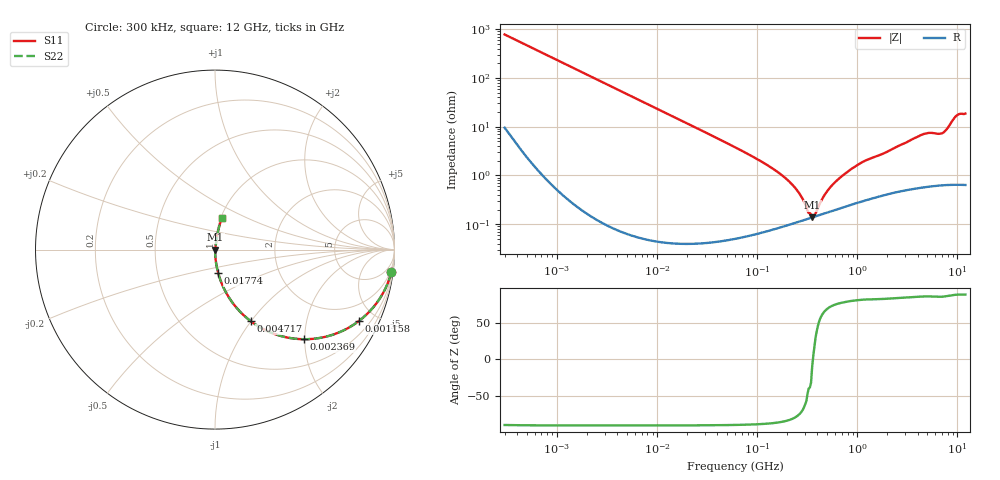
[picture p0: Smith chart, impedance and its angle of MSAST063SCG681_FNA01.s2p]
! MSAST063SCG681_FNA01  S-PARAMETER MODEL  ( General Type )
! Model Generated by TAIYO YUDEN Corporation (http://www.ty-top.com)
! Version 1.0
! TAIYO YUDEN Control No. 160830
! Copyright(c) 2016 TAIYO YUDEN CO.,LTD. All Rights Reserved.
! Product Description (link to TY-COMPAS)
! https://ds.yuden.co.jp/TYCOMPAS/or/detail?pn=MSAST063SCG681JFNA01&u=M
! Products Name : Multilayer Ceramic Capacitors
! Characteristics :
!  Capacitance : 680 pF , Rated Voltage : 25V , TCC : CG / C0G
!  Case Size : 0.6 x 0.3 / 0.024 x 0.012 [mm/inch] , Thickness : 0.3 / 0.012 [mm/inch]
!  (Conditions: Temperature = 25 degC , DC Bias Current/Voltage = 0A / 0V)
! External Node Assignments :
!  1  o---| |---o  2
! GND o---------o GND
! Frequency Range : 0.3MHz  -  12000MHz  [ 401 STEP ]
# MHz S RI R 50
! Freq[MHz].  S11 Real  S11 Imag  S21 Real  S21 Imag  S12 Real  S12 Imag  S22 Real  S22 Imag
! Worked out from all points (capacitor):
!   401 points, 300 kHz to 12 GHz, reference 50 ohm
!   read as one part in series: C = 680 pF near 316.3 kHz
!   lowest |Z| = 140 mohm at 354 MHz (marker M1)
!   series resonance near 360.2 MHz, so ESL is about 290 pH
!   S11 on the Smith chart (normalised r, x): 300 kHz: 1, -16; 1.158 MHz: 1.01, -4.04; 2.369 MHz: 1.00, -1.98; 4.717 MHz: 1.00, -0.99; 17.74 MHz: 1.00, -0.26; 12 GHz: 1.01, +0.37
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0.3  0.9823 -0.1257  0.0177 0.1257  0.0177 0.1257  0.9823 -0.1257
0.646801  0.9283 -0.2563  0.0717 0.2563  0.0717 0.2563  0.9283 -0.2563
1.158468  0.8028 -0.397  0.1972 0.397  0.1972 0.397  0.8028 -0.397
1.769972  0.636 -0.4804  0.364 0.4804  0.364 0.4804  0.636 -0.4804
2.36877  0.494 -0.4993  0.506 0.4993  0.506 0.4993  0.494 -0.4993
4.716902  0.1978 -0.3977  0.8022 0.3977  0.8022 0.3977  0.1978 -0.3977
10.44266  0.0481 -0.2131  0.9519 0.2131  0.9519 0.2131  0.0481 -0.2131
17.7384  0.0174 -0.1293  0.9826 0.1293  0.9826 0.1293  0.0174 -0.1293
60  0.00193 -0.0378  0.9981 0.0378  0.9981 0.0378  0.00193 -0.0378
197.6437  0.00101 -0.00825  0.999 0.00825  0.999 0.00825  0.00101 -0.00825
257.5933  0.00113 -0.00442  0.9989 0.00442  0.9989 0.00442  0.00113 -0.00442
335.7268  0.00133 -0.00105  0.9987 0.00105  0.9987 0.00105  0.00133 -0.00105
353.9943  0.00137 -0.000237  0.9986 0.000237  0.9986 0.000237  0.00137 -0.000237
383.2761  0.00145 0.000845  0.9985 -0.000845  0.9985 -0.000845  0.00145 0.000845
499.5319  0.00175 0.0044  0.9982 -0.0044  0.9982 -0.0044  0.00175 0.0044
668.5285  0.00218 0.00864  0.9978 -0.00864  0.9978 -0.00864  0.00218 0.00864
1105.905  0.00324 0.0181  0.9968 -0.0181  0.9968 -0.0181  0.00324 0.0181
2088.533  0.00518 0.0317  0.9948 -0.0317  0.9948 -0.0317  0.00518 0.0317
4502.883  0.0103 0.0683  0.9897 -0.0683  0.9897 -0.0683  0.0103 0.0683
7064.448  0.0115 0.0722  0.9885 -0.0722  0.9885 -0.0722  0.0115 0.0722
9708.23  0.0327 0.1596  0.9673 -0.1596  0.9673 -0.1596  0.0327 0.1596
12000  0.0391 0.1774  0.9609 -0.1774  0.9609 -0.1774  0.0391 0.1774
